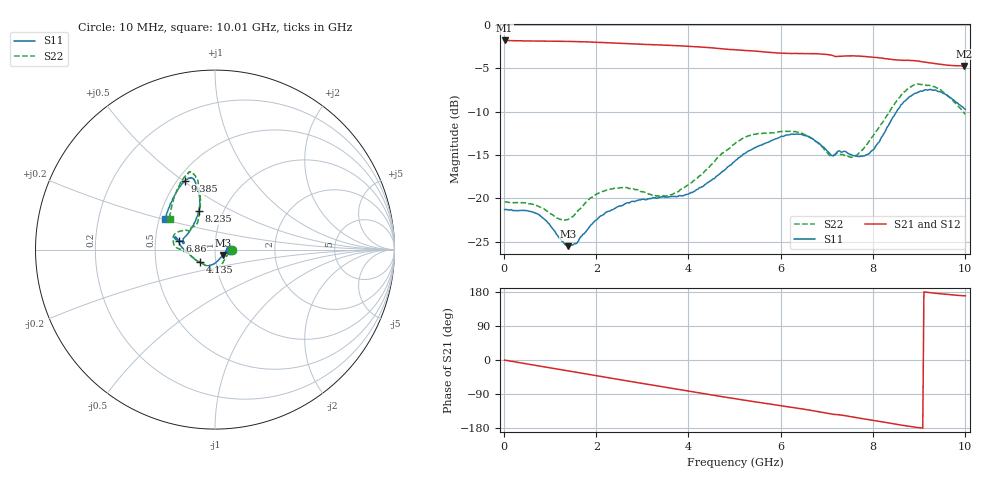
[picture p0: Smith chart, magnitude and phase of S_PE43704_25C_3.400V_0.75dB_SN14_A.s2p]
! Device ID: PE43704
! Dir: z:\PE43704\PE43704_Char_1_20130516\PE43704\AMB\3p400V\0p75dB
! Serial: 14
! Insertion: A
! Impedance: 50 ohm
! Temp: Amb
! VDD: 3.400V
! Attenuation Step: 0.75dB
! IDD: 1.140682e-01mA
#  Hz  S  RI  R  50
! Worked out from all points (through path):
!   401 points, 10 MHz to 10.01 GHz, reference 50 ohm
!   highest |S21| = -1.79 dB at 10 MHz (marker M1); lowest = -4.7 dB at 9.985 GHz (marker M2)
!   group delay of S21, straight-line fit = 54.2 ps
!   lowest |S11| = -25.5 dB at 1.385 GHz (marker M3), VSWR 1.11, Z = 54.5 - j3.25 ohm
!   |S11| at or under -10 dB: start of sweep to 8.517 GHz
!   |S22| runs from -22.5 to -6.8 dB; largest |S21 - S12| = 0.0058
!   S11 on the Smith chart (normalised r, x): 10 MHz: 1.19, +0.00; 4.135 GHz: 0.84, -0.12; 6.86 GHz: 0.67, +0.07; 8.235 GHz: 0.76, +0.35; 9.385 GHz: 0.55, +0.51; 10.01 GHz: 0.54, +0.21
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1e7  0.0861 0.000178  0.8139 -0.00324  0.8138 -0.00307  0.0955 0.000124
7.35e8  0.0797 0.0155  0.7792 -0.2123  0.7792 -0.2121  0.0899 0.00687
1.385e9  0.0438 -0.0298  0.7046 -0.387  0.7045 -0.387  0.0581 -0.0483
1.685e9  0.0219 -0.0566  0.6551 -0.4598  0.6551 -0.4598  0.0368 -0.0809
2.385e9  -0.0197 -0.0847  0.5114 -0.5975  0.5117 -0.5972  -0.01 -0.1139
3.36e9  -0.0441 -0.0909  0.2746 -0.716  0.2752 -0.7156  -0.0502 -0.0898
4.135e9  -0.0846 -0.0701  0.0692 -0.746  0.0696 -0.7465  -0.1182 -0.0476
5.01e9  -0.1642 -0.0056  -0.1501 -0.7032  -0.1498 -0.7036  -0.2069 0.00646
5.385e9  -0.1909 0.0219  -0.2342 -0.6683  -0.2341 -0.6688  -0.2302 0.0322
6.085e9  -0.2188 0.0695  -0.362 -0.5835  -0.3596 -0.5831  -0.233 0.0717
6.685e9  -0.2145 0.0545  -0.4704 -0.4954  -0.4708 -0.4943  -0.196 0.1024
6.86e9  -0.1988 0.0495  -0.4994 -0.4631  -0.5012 -0.4625  -0.1721 0.1071
7.085e9  -0.1736 0.0431  -0.5284 -0.414  -0.5308 -0.4144  -0.1445 0.1002
7.585e9  -0.1549 0.0835  -0.5796 -0.3232  -0.5784 -0.3227  -0.1017 0.1421
7.91e9  -0.1223 0.1323  -0.6043 -0.2509  -0.6063 -0.254  -0.0891 0.1918
8.235e9  -0.0919 0.2162  -0.6172 -0.1791  -0.6164 -0.1827  -0.0814 0.2681
8.36e9  -0.0849 0.2555  -0.6169 -0.1492  -0.6169 -0.1529  -0.0825 0.3049
8.835e9  -0.1099 0.3737  -0.6222 -0.0433  -0.6182 -0.0459  -0.121 0.4226
9.385e9  -0.168 0.3829  -0.5954 0.0435  -0.5963 0.0462  -0.1761 0.3956
9.66e9  -0.2157 0.3186  -0.5802 0.0777  -0.5771 0.0789  -0.2173 0.3153
9.985e9  -0.2724 0.1842  -0.5698 0.106  -0.5723 0.1087  -0.2505 0.1814
1.001e10  -0.2778 0.1712  -0.5712 0.1082  -0.5745 0.1092  -0.253 0.1716
